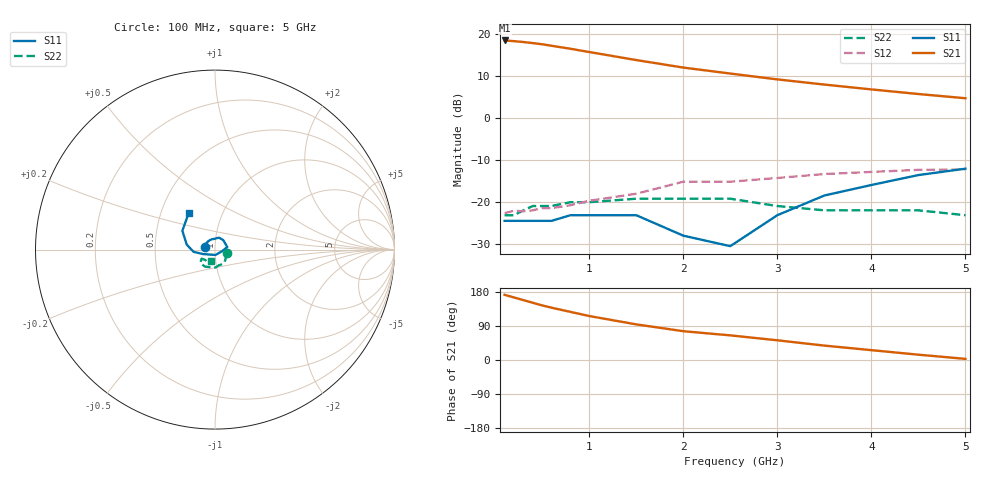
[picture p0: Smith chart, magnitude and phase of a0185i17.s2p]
!  MSA-0185 S AND NOISE PARAMETERS
!  Id=17mA  LAST UPDATED 07-22-92
# ghz s ma r 50
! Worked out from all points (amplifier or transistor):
!   16 points, 100 MHz to 5 GHz, reference 50 ohm
!   highest |S21| = 18.4 dB at 100 MHz (marker M1)
!   |S21| within 3 dB of that: start of sweep to 1.065 GHz
!   unconditionally stable (mu >= 1): start of sweep to end of sweep
!   at 300 MHz: K = 1.10, MAG = 18.2 dB, |S12| = -22.2 dB
!   at 1.5 GHz: K = 1.11, MAG = 13.9 dB, |S12| = -18.0 dB
!   at 5 GHz: K = 1.30, MAG = 5.2 dB, |S12| = -12.2 dB
!   lowest NFmin = 5.20 dB at 100 MHz
0.1  0.06 166.0  8.36 172.0  0.074 3.0  0.07 -17.0
0.2  0.06 149.0  8.2 165.0  0.079 8.0  0.07 -28.0
0.3  0.06 133.0  8.01 158.0  0.078 11.0  0.08 -43.0
0.4  0.06 120.0  7.78 151.0  0.08 14.0  0.09 -56.0
0.5  0.06 105.0  7.53 144.0  0.085 18.0  0.09 -68.0
0.6  0.06 94.0  7.23 138.0  0.085 19.0  0.09 -75.0
0.8  0.07 72.0  6.66 127.0  0.092 24.0  0.1 -89.0
1  0.07 49.0  6.09 116.0  0.104 27.0  0.1 -100.0
1.5  0.07 12.0  4.89 94.0  0.126 32.0  0.11 -120.0
2  0.04 -13.0  3.98 76.0  0.175 31.0  0.11 -134.0
2.5  0.03 -84.0  3.38 65.0  0.175 33.0  0.11 -138.0
3  0.07 -159.0  2.88 52.0  0.194 29.0  0.09 -146.0
3.5  0.12 -174.0  2.5 38.0  0.216 24.0  0.08 -135.0
4  0.16 170.0  2.19 26.0  0.229 19.0  0.08 -120.0
4.5  0.21 150.0  1.93 14.0  0.242 13.0  0.08 -107.0
5  0.25 126.0  1.72 3.0  0.245 -6.0  0.07 -110.0
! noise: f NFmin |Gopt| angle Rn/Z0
0.1  5.2  0.23  2  1.13
0.5  5.3  0.23  7  1.12
1  5.5  0.21  13  1.1
2  5.8  0.18  26  1.04
